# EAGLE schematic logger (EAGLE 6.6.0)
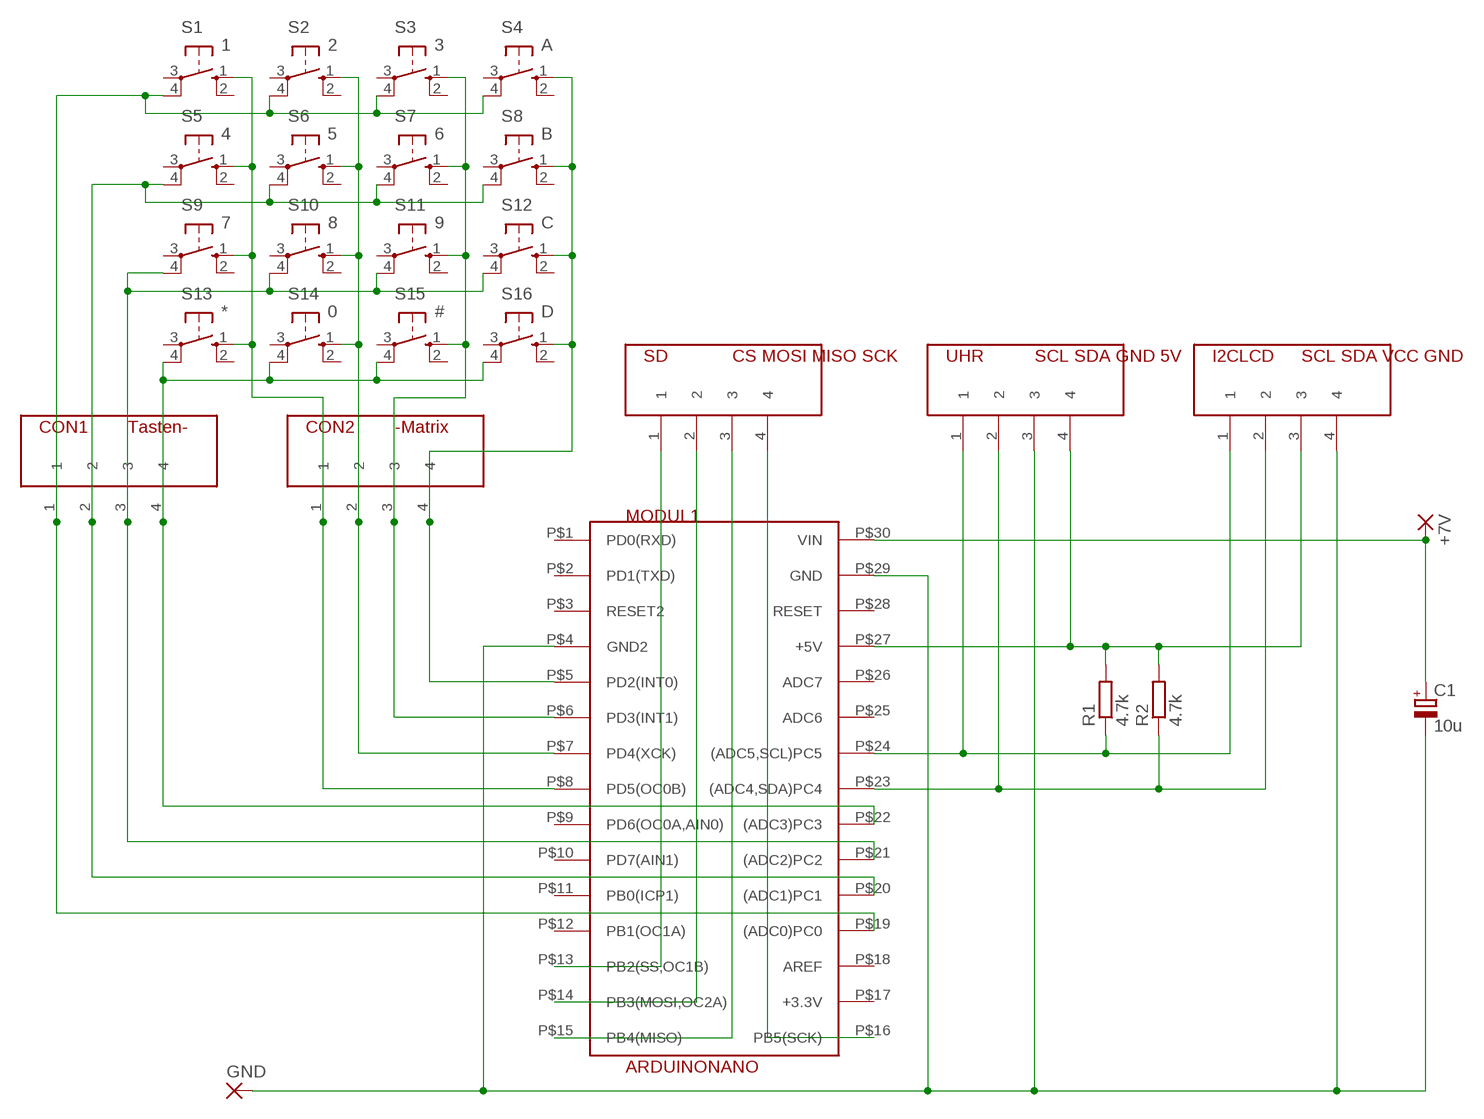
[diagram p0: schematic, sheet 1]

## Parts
+7V  1,6/0,8  [1,6/0,8]
C1  10u  CPOL-EUE7.5-16  [E7,5-16]
CON1  Tasten-  4POL-STECKERN  [STECKER4]
CON2  -Matrix  4POL-STECKERN  [STECKER4]
GND  1,6/0,8  [1,6/0,8]
I2CLCD  SCL SDA VCC GND  4POL-STECKERN  [STECKER4]
MODUL1  ARDUINONANO  [ARDUINONANO]
R1  4.7k  R-EU_0204/7  [0204/7]
R2  4.7k  R-EU_0204/7  [0204/7]
S1  1  10-XX  [B3F-10XX]
S2  2  10-XX  [B3F-10XX]
S3  3  10-XX  [B3F-10XX]
S4  A  10-XX  [B3F-10XX]
S5  4  10-XX  [B3F-10XX]
S6  5  10-XX  [B3F-10XX]
S7  6  10-XX  [B3F-10XX]
S8  B  10-XX  [B3F-10XX]
S9  7  10-XX  [B3F-10XX]
S10  8  10-XX  [B3F-10XX]
S11  9  10-XX  [B3F-10XX]
S12  C  10-XX  [B3F-10XX]
S13  *  10-XX  [B3F-10XX]
S14  0  10-XX  [B3F-10XX]
S15  #  10-XX  [B3F-10XX]
S16  D  10-XX  [B3F-10XX]
SD  CS MOSI MISO SCK  4POL-STECKERN  [STECKER4]
UHR  SCL SDA GND 5V  4POL-STECKERN  [STECKER4]

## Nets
GND: C1.- GND.1(P) I2CLCD.4 MODUL1.P$4(GND2) MODUL1.P$29(GND) UHR.3
N$1: I2CLCD.1 MODUL1.P$24((ADC5,SCL)PC5) R1.1 UHR.1
N$3: I2CLCD.2 MODUL1.P$23((ADC4,SDA)PC4) R2.1 UHR.2
N$4: MODUL1.P$13(PB2(SS,OC1B)) SD.1
N$5: MODUL1.P$14(PB3(MOSI,OC2A)) SD.2
N$6: MODUL1.P$15(PB4(MISO)) SD.3
N$7: MODUL1.P$16(PB5(SCK)) SD.4
N$9: CON2.3 MODUL1.P$6(PD3(INT1)) S3.1(S) S7.1(S) S11.1(S) S15.1(S)
N$10: CON2.2 MODUL1.P$7(PD4(XCK)) S2.1(S) S6.1(S) S10.1(S) S14.1(S)
N$11: CON2.1 MODUL1.P$8(PD5(OC0B)) S1.1(S) S5.1(S) S9.1(S) S13.1(S)
N$12: CON1.4 MODUL1.P$22((ADC3)PC3) S13.4(P1) S14.4(P1) S15.4(P1) S16.4(P1)
N$13: CON2.4 MODUL1.P$5(PD2(INT0)) S4.1(S) S8.1(S) S12.1(S) S16.1(S)
N$15: CON1.3 MODUL1.P$21((ADC2)PC2) S9.4(P1) S10.4(P1) S11.4(P1) S12.4(P1)
N$16: CON1.2 MODUL1.P$20((ADC1)PC1) S5.4(P1) S6.4(P1) S7.4(P1) S8.4(P1)
N$17: CON1.1 MODUL1.P$19((ADC0)PC0) S1.4(P1) S2.4(P1) S3.4(P1) S4.4(P1)
VDD: I2CLCD.3 MODUL1.P$27(+5V) R1.2 R2.2 UHR.4
VIN: +7V.1(P) C1.+ MODUL1.P$30(VIN)
Unconnected: MODUL1.P$1(PD0(RXD)) MODUL1.P$2(PD1(TXD)) MODUL1.P$3(RESET2) MODUL1.P$9(PD6(OC0A,AIN0)) MODUL1.P$10(PD7(AIN1)) MODUL1.P$11(PB0(ICP1)) MODUL1.P$12(PB1(OC1A)) MODUL1.P$17(+3.3V) MODUL1.P$18(AREF) MODUL1.P$25(ADC6) MODUL1.P$26(ADC7) MODUL1.P$28(RESET) S1.2(S1) S1.3(P) S2.2(S1) S2.3(P) S3.2(S1) S3.3(P) S4.2(S1) S4.3(P) S5.2(S1) S5.3(P) S6.2(S1) S6.3(P) S7.2(S1) S7.3(P) S8.2(S1) S8.3(P) S9.2(S1) S9.3(P) S10.2(S1) S10.3(P) S11.2(S1) S11.3(P) S12.2(S1) S12.3(P) S13.2(S1) S13.3(P) S14.2(S1) S14.3(P) S15.2(S1) S15.3(P) S16.2(S1) S16.3(P)

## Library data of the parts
+7V GND = wirepad:1,6/0,8: THROUGH-HOLE PAD
C1 = rcl:CPOL-EU: POLARIZED CAPACITOR, European symbol
CON1 CON2 I2CLCD SD UHR = 6_stecker:4POL-STECKER
MODUL1 = arduino:ARDUINONANO
R1 R2 = resistor:R-EU_: RESISTOR, European symbol
S1-S16 = switch-omron:10-XX: OMRON SWITCH; MPN: B3F-1000; OC_FARNELL: 176432; OC_NEWARK: 36M3542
